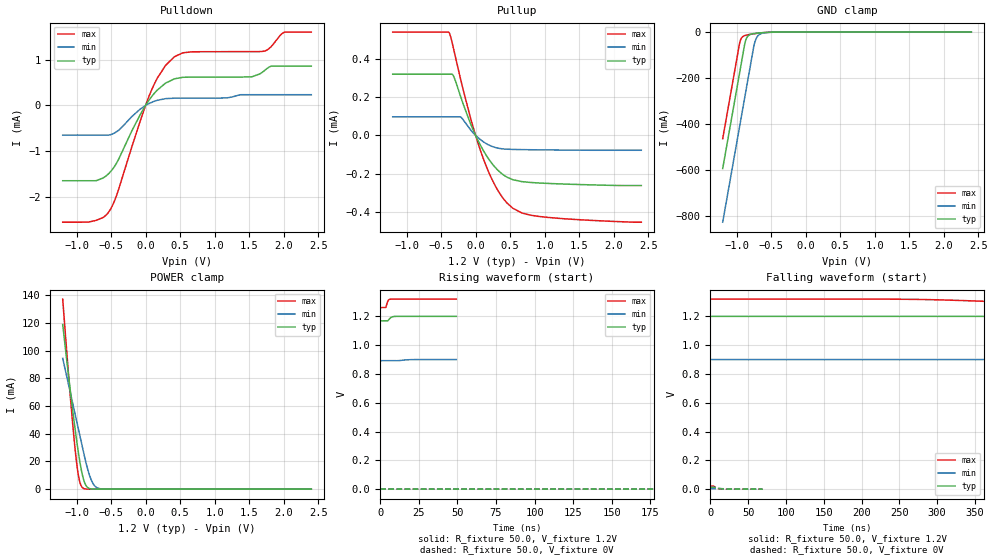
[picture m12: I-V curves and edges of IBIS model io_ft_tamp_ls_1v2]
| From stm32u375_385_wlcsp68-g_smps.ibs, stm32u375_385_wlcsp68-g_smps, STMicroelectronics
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[Model]   io_ft_tamp_ls_1v2
Model_type I/O
Polarity   Non-Inverting
Enable   Active-Low
| CAP_THRESHOLD on pad IOFT is "UDTCAPC" :
| Rising=30.0% of vddios   Falling=70.0% of vddios
| C_comp min and max val. don't necessarily correlate with the min and max pvt
| but are the smallest and greatest pad capacitance found.
| var   typ   min   max
C_comp   2.41252pF  2.38312pF  2.43304pF
|C_comp_pullup   1.39440pF  1.29315pF  1.47713pF
|C_comp_pulldown   1.01813pF  1.08997pF  955.90639fF
Vinl = 450.0mV
Vinh = 660.0mV
Vmeas = 600.0mV   | Reference voltage for timing measurements
Cref  = 50.0pF   | Timing specification test load capacitance value
Rref  = 1.0MOhm   | Timing specification test load resistance value
Vref  = 660.0mV   | Timing specification test load voltage
[Model Spec]
| TIME_THRESHOLD on pin ZIV11 is "CMOS" :
| Rising=50.0% of vdd   Falling=50.0% of vdd
Vinl 439.50000mV 331.50001mV 485.50000mV
Vinh 752.50000mV 552.50001mV 837.50000mV
| variable   typ   min   max
[Temperature Range] 25.0 130.0 -40.0
| variable   typ   min   max
[Voltage Range] 1.2V 900.0mV 1.32V
| variable   typ   min   max
[POWER Clamp Reference] 1.2V 900.0mV 1.32V
| variable   typ   min   max
[GND Clamp Reference] 0V 0V 0V
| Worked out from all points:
|   slope of the pulldown table from 0 to 0.18 V, typ, clamps not added: 514 ohm
|   slope of the pullup table from 0 to 0.18 V, typ, clamps not added: 1.52 kohm
|   GND clamp passes 1 mA (typ) near -0.53 V on its own axis
|   POWER clamp passes 1 mA (typ) near -0.83 V on its own axis
[POWER Clamp]
-1.2V     118.8mA    94.44mA    137.2mA
-1.09V    71.2mA     69.75mA    67.14mA
-1.02V    43.22mA    54.03mA    28.67mA
-990mV    32.26mA    47.3mA     15.78mA
-970mV    25.49mA    42.81mA    9.257mA
-940mV    16.45mA    36.08mA    3.257mA
-910mV    9.238mA    29.34mA    904.6uA
-860mV    2.387mA    18.53mA    87.46uA
-790mV    204.6uA    7.049mA    3.101uA
-730mV    21.91uA    2.041mA    176.4nA
-660mV    1.594uA    337.6uA    6.258nA
2.4V      0A         0A         0A
[GND Clamp]
-1.2V     -593.4mA   -826.9mA   -463.7mA
-960mV    -185.4mA   -418.9mA   -55.68mA
-940mV    -151.4mA   -384.9mA   -33.02mA
-880mV    -50.24mA   -282.9mA   -15.1mA
-850mV    -23.55mA   -231.9mA   -12.72mA
-810mV    -11.44mA   -163.9mA   -10.41mA
-740mV    -5.957mA   -49.45mA   -7.062mA
-710mV    -4.858mA   -24.97mA   -5.804mA
-670mV    -3.677mA   -10.87mA   -4.301mA
-590mV    -1.88mA    -3mA       -1.97mA
-390mV    -51.73uA   -182.4uA   -18.95uA
2.4V      708.1pA    117.2nA    245.1pA
| variable   typ   min   max
[Pullup Reference] 1.2V 900.0mV 1.32V
| variable   typ   min   max
[Pulldown Reference] 0V 0V 0V
[Pullup]
-1.2V     320.5uA    97.29uA    541.3uA
-380mV    320.5uA    97.29uA    536.6uA
-320mV    311.1uA    97.29uA    456uA
-210mV    196.5uA    94.51uA    284.2uA
-50mV     41.04uA    19.26uA    61.66uA
100mV     -71.38uA   -30.42uA   -109.8uA
210mV     -134.4uA   -53.59uA   -209.2uA
320mV     -181.6uA   -66.67uA   -287uA
540mV     -232.4uA   -73.77uA   -382.1uA
670mV     -242.4uA   -74.73uA   -406.8uA
1.04V     -251.8uA   -76.3uA    -429.8uA
2.4V      -263.1uA   -78.1uA    -455.1uA
[Pulldown]
-1.2V     -1.647mA   -647.5uA   -2.554mA
-730mV    -1.647mA   -647.5uA   -2.52mA
-530mV    -1.485mA   -646.3uA   -2.323mA
-420mV    -1.261mA   -574.3uA   -1.968mA
80mV      177.8uA    62.73uA    313.5uA
290mV     489.8uA    149.3uA    878.6uA
420mV     583.8uA    159.3uA    1.068mA
670mV     620.6uA    160uA      1.174mA
1.54V     627.5uA    235.2uA    1.177mA
1.71V     748.6uA    235.2uA    1.186mA
2.01V     861.2uA    235.2uA    1.602mA
2.4V      861.2uA    235.2uA    1.605mA
[Ramp]
dV/dt_r 7.6175mV/399.16844ns 2.26826mV/1.02415us 13.12387mV/218.92256ns
dV/dt_f 18.65902mV/386.59526ns 4.79954mV/1.04073us 35.31781mV/227.5729ns
R_load = 50.0
| Removed startup time: 0s 0s 0s  .
| Removed end time: 49.25ns.
[Rising Waveform]
R_fixture   = 50.0
V_fixture   = 1.2V
V_fixture_min = 900.0mV
V_fixture_max = 1.32V
0s        1.169V     892mV      1.261V
3.5ns     1.169V     892mV      1.261V
3.75ns    1.169V     892mV      1.266V
5.05ns    1.171V     892mV      1.309V
5.7ns     1.179V     892mV      1.317V
6.45ns    1.188V     892mV      1.319V
8.05ns    1.197V     892mV      1.32V
10.05ns   1.2V       892mV      1.32V
21.15ns   1.2V       899.4mV    1.32V
49.25ns   1.2V       900mV      1.32V
| Removed startup time: 0s 0s 0s  .
| Removed end time: 5.4992us.
[Falling Waveform]
R_fixture   = 50.0
V_fixture   = 1.2V
V_fixture_min = 900.0mV
V_fixture_max = 1.32V
0s        1.2V       900mV      1.32V
272.2ns   1.2V       900mV      1.318V
497.8ns   1.198V     900mV      1.281V
561.2ns   1.196V     900mV      1.274V
656.4ns   1.191V     900mV      1.267V
820.4ns   1.182V     900mV      1.263V
1.122us   1.172V     900mV      1.261V
1.571us   1.169V     899.2mV    1.261V
3.143us   1.169V     892.8mV    1.261V
5.499us   1.169V     892mV      1.261V
| Removed startup time: 0s 0s 0s  .
| Removed end time: 5.4992us.
[Rising Waveform]
R_fixture   = 50.0
V_fixture   = 0V
V_fixture_min = 0V
V_fixture_max = 0V
0s        10.41nV    204nV      9.892nV
112.2ns   -4.871uV   -937.9nV   -4.086uV
224.4ns   4.885uV    -887.3nV   3.577mV
336.6ns   434.4uV    -707.7nV   11.72mV
468.2ns   2.967mV    71.94nV    17.95mV
606.2ns   6.208mV    3.153uV    20.58mV
785.6ns   9.383mV    13.16uV    21.56mV
1.459us   12.52mV    1.023mV    21.86mV
2.694us   12.69mV    3.34mV     21.87mV
5.499us   12.7mV     3.781mV    21.87mV
| Removed startup time: 0s 0s 0s  .
| Removed end time: 69.2ns.
[Falling Waveform]
R_fixture   = 50.0
V_fixture   = 0V
V_fixture_min = 0V
V_fixture_max = 0V
0s        12.7mV     3.79mV     21.88mV
4.2ns     12.7mV     3.79mV     21.88mV
5.45ns    12.63mV    3.79mV     17.74mV
7.8ns     9.595mV    3.789mV    10.41mV
10.2ns    6.794mV    3.792mV    4.604mV
12.05ns   4.905mV    3.802mV    1.703mV
14.8ns    2.603mV    3.498mV    341.7uV
22.6ns    170.1uV    2.263mV    70.51uV
42.4ns    15.16uV    297.6uV    2.045uV
69.2ns    879.3nV    23.58uV    1.188uV
